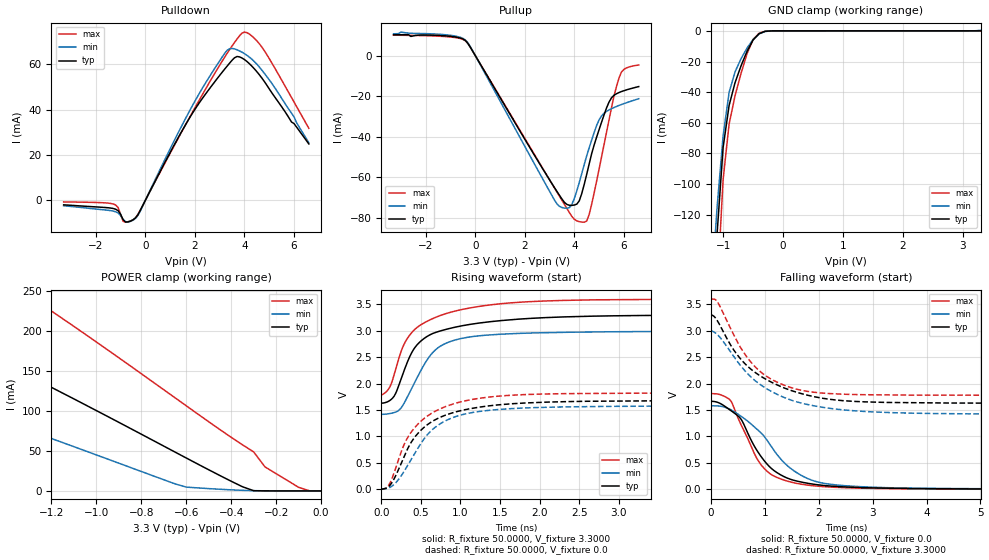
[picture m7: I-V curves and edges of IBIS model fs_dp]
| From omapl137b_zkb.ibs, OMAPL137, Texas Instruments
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|   Model fs_dp
[Model]   fs_dp
Model_type   3-state
Polarity   Non-Inverting
Enable   Active-Low
Vmeas =   1.5000V
C_comp   5.0000pF   5.0000pF   5.0000pF
[Temperature Range]   25.0000   0.1100k   -40.0000
[Voltage Range]   3.3000V   3.0000V   3.6000V
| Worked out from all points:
|   slope of the pulldown table from 0 to 0.495 V, typ, clamps not added: 46.8 ohm
|   slope of the pullup table from 0 to 0.495 V, typ, clamps not added: 48.3 ohm
|   GND clamp passes 1 mA (typ) near -0.35 V on its own axis
|   POWER clamp passes 1 mA (typ) near -0.31 V on its own axis
|   rising waveform, R_fixture 50.0000, V_fixture 3.3000: 20-80 % time 460ps typ, 395ps min, 500ps max; typ from 1.63 V to 3.3 V
|   rising waveform, R_fixture 50.0000, V_fixture 0.0: 20-80 % time 512ps typ, 495ps min, 483ps max; typ from 0 V to 1.68 V
|   falling waveform, R_fixture 50.0000, V_fixture 0.0: 20-80 % time 643ps typ, 874ps min, 554ps max; typ from 1.67 V to 0.001 V
|   falling waveform, R_fixture 50.0000, V_fixture 3.3000: 20-80 % time 1.02ns typ, 1.06ns min, 751ps max; typ from 3.3 V to 1.63 V
[Pulldown]
|Voltage   I(typ)   I(min)   I(max)
-3.3V     -2.015mA   -2.423mA   -731.2uA
-1.3V     -3.626mA   -4.772mA   -1.634mA
-1.1V     -4.613mA   -5.62mA    -3.221mA
-900mV    -8.569mA   -8.416mA   -9.25mA
-400mV    -7.775mA   -7.992mA   -7.73mA
1.7V      34.77mA    37.67mA    34.83mA
3.1V      56.44mA    63.16mA    61.32mA
3.3V      59.14mA    66.09mA    64.75mA
3.6V      62.82mA    66.74mA    69.58mA
4V        62.02mA    64.63mA    74.14mA
4.8V      52.4mA     56mA       65.98mA
6.6V      24.82mA    25.34mA    31.71mA
[Pullup]
|Voltage   I(typ)   I(min)   I(max)
-3.3V     10.22mA    10.72mA    10.04mA
-400mV    7.43mA     7.696mA    7.269mA
3.3V      -67.08mA   -73.18mA   -67.35mA
3.8V      -73.86mA   -75mA      -77.45mA
4.1V      -73.3mA    -66.74mA   -81.55mA
4.3V      -68.08mA   -58.24mA   -82.13mA
4.6V      -53.44mA   -45.5mA    -78.36mA
5V        -36.54mA   -31.71mA   -56mA
5.4V      -22.98mA   -26.84mA   -31.82mA
5.8V      -18.27mA   -24.65mA   -11.23mA
6V        -17.35mA   -23.74mA   -6.838mA
6.6V      -15.31mA   -21.31mA   -4.665mA
[GND_clamp]
|Voltage   I(typ)   I(min)   I(max)
-3.3V     -2.102A    -1.576A    -3.228A
-1.2V     -207.9mA   -171.6mA   -289.7mA
-1.1V     -132.1mA   -115mA     -169.9mA
-1V       -76.03mA   -68.46mA   -96.96mA
-900mV    -48.63mA   -40.12mA   -60.78mA
-800mV    -33.68mA   -26.64mA   -42.17mA
-700mV    -22.71mA   -18.11mA   -27.61mA
-600mV    -13.24mA   -11.16mA   -14.78mA
-500mV    -5.931mA   -5.609mA   -5.62mA
-400mV    -1.814mA   -2.008mA   -1.538mA
-200mV    -13.57uA   -34.99uA   -6.398uA
3.3V      27.63uA    374.3uA    27.55uA
[POWER_clamp]
|Voltage   I(typ)   I(min)   I(max)
-3.3V     434.5mA    862.7mA    595.9mA
-2.35V    281.5mA    249.7mA    422.2mA
-2.2V     262.7mA    179.3mA    401.4mA
-2.1V     250.3mA    155mA      385.4mA
-2V       237.7mA    143.8mA    368.9mA
-1.3V     143.6mA    75.64mA    243.6mA
-600mV    41.12mA    4.791mA    106.3mA
-350mV    5.253mA    778.4uA    57.63mA
-300mV    274.5uA    374.3uA    48.71mA
-250mV    91.11uA    154.3uA    30.09mA
-100mV    28.77uA    28.48uA    4.516mA
0V        27.63uA    25.47uA    25.47uA
[Ramp]
| variable   typ   min   max
dV/dt_r   1.0075/0.5119n   0.9492/0.4952n   1.0921/0.4834n
dV/dt_f   1.0025/1.0170n   0.9483/1.0559n   1.0919/0.7508n
R_load =   50.0000
[Rising Waveform]
R_fixture=   50.0000
V_fixture=   3.3000
V_fixture_min=  3.0000
V_fixture_max=  3.6000
|time   V(typ)   V(min)   V(max)
0s        1.628V     1.415V     1.779V
99.1ps    1.67V      1.429V     1.911V
162.2ps   1.76V      1.45V      2.165V
288.3ps   2.245V     1.626V     2.745V
441.4ps   2.714V     2.079V     3.049V
603.6ps   2.913V     2.502V     3.197V
747.7ps   2.996V     2.708V     3.289V
1.315ns   3.16V      2.914V     3.477V
3.054ns   3.284V     2.982V     3.59V
9ns       3.299V     2.997V     3.599V
[Rising Waveform]
R_fixture=   50.0000
V_fixture=   0.0
V_fixture_min=  0.0
V_fixture_max=  0.0
|time   V(typ)   V(min)   V(max)
0s        1.555uV    4.781uV    1.371uV
99.1ps    55.17mV    25.62mV    86.41mV
198.2ps   305.5mV    147.1mV    473.4mV
324.3ps   737.4mV    426.6mV    953.4mV
504.5ps   1.121V     874.9mV    1.292V
639.6ps   1.279V     1.12V      1.44V
801.8ps   1.396V     1.287V     1.558V
1.27ns    1.56V      1.477V     1.727V
2.766ns   1.667V     1.566V     1.815V
9ns       1.679V     1.582V     1.82V
[Falling Waveform]
R_fixture=   50.0000
V_fixture=   0.0
V_fixture_min=  0.0
V_fixture_max=  0.0
|time   V(typ)   V(min)   V(max)
0s        1.666V     1.581V     1.811V
360.4ps   1.493V     1.507V     1.68V
558.6ps   1.321V     1.38V      1.214V
828.8ps   769.6mV    1.156V     621.3mV
991ps     533mV      993.1mV    386.6mV
1.306ns   262.9mV    555.4mV    189mV
1.595ns   153.3mV    309.8mV    108.9mV
2.063ns   73.7mV     117.2mV    50.23mV
2.973ns   24.87mV    38.35mV    15.2mV
9ns       1.267mV    3.785mV    515.7uV
[Falling Waveform]
R_fixture=   50.0000
V_fixture=   3.3000
V_fixture_min=  3.0000
V_fixture_max=  3.6000
|time   V(typ)   V(min)   V(max)
0s        3.299V     2.999V     3.599V
117.1ps   3.188V     2.927V     3.548V
459.5ps   2.58V      2.458V     2.845V
630.6ps   2.374V     2.239V     2.551V
828.8ps   2.203V     2.046V     2.306V
1.189ns   1.992V     1.814V     2.045V
1.685ns   1.808V     1.628V     1.872V
2.351ns   1.686V     1.513V     1.803V
3.459ns   1.64V      1.446V     1.783V
9ns       1.629V     1.419V     1.779V
